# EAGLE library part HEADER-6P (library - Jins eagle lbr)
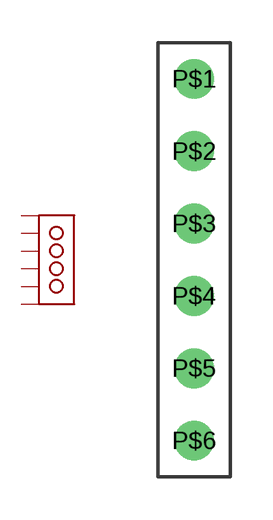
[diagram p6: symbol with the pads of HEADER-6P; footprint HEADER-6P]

Designator prefix H

## HEADER-6P  [HEADER-6P]
P$1  P$1
P$2  P$2
P$3  P$3
P$4  P$4
P$5  P$5
P$6  P$6

## Footprint HEADER-6P (pad centres in mm)
drill 0.8 pad 1.4: P$1 0,2.54; P$2 0,0; P$3 0,-2.54; P$4 0,-5.08; P$5 0,-7.62; P$6 0,-10.16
